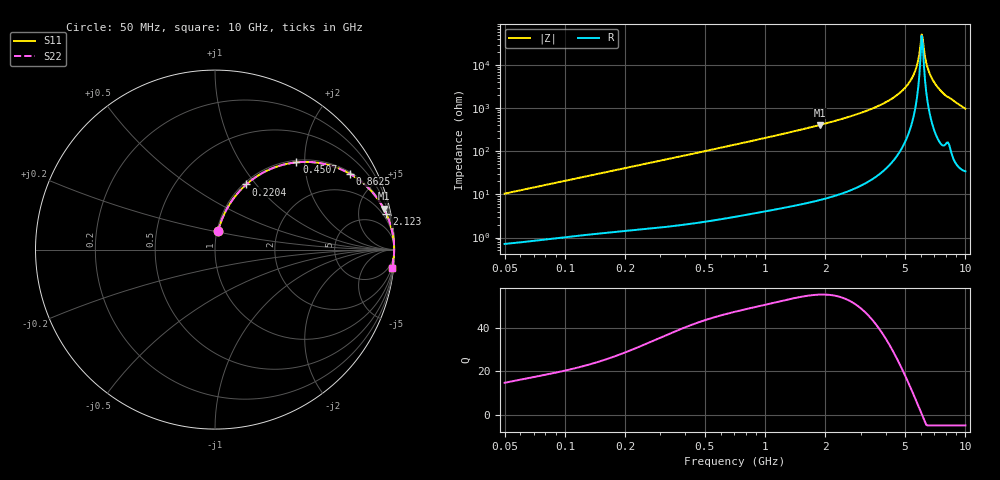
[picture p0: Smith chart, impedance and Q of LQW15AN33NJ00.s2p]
!Murata Part Number: LQW15AN33NJ00
!These Parameters are Measured in Series Mode Connection
!  o--[Z]--o
!Port1  Port2
!  o-------o
!Freq. Start=50[MHz] Stop=10[GHz], 401[Steps]
# Hz S RI R 50
!Freq.(Hz)	S 11(Real)	S 11(Imag)	S 21(Real)	S 21(Imag)	S 12(Real)	S 12(Imag)	S 22(Real)	S 22(Imag)
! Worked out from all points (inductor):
!   401 points, 50 MHz to 10 GHz, reference 50 ohm
!   read as one part in series: L = 33 nH near 51.34 MHz
!   highest Q = 55.3 at 1.884 GHz (marker M1), where L = 34.7 nH
!   self-resonance near 6.045 GHz
!   S11 on the Smith chart (normalised r, x): 50 MHz: 1.01, +0.21; 220.4 MHz: 1.03, +0.89; 450.7 MHz: 1.04, +1.82; 862.5 MHz: 1.07, +3.51; 2.123 GHz: 1.17, +9.53; 10 GHz: 2, -20
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5e7  0.0175 0.1015  0.9825 -0.1015  0.9825 -0.1015  0.0175 0.1015
1.214486e8  0.0673 0.2291  0.9327 -0.2291  0.9327 -0.2291  0.0673 0.2291
2.204238e8  0.1742 0.3631  0.8258 -0.3631  0.8258 -0.3631  0.1742 0.3631
2.949953e8  0.2678 0.4288  0.7322 -0.4288  0.7322 -0.4288  0.2678 0.4288
4.507103e8  0.4536 0.4861  0.5464 -0.4861  0.5464 -0.4861  0.4536 0.4861
7.071068e8  0.6686 0.4603  0.3314 -0.4603  0.3314 -0.4603  0.6686 0.4603
8.625288e8  0.7502 0.4229  0.2498 -0.4229  0.2498 -0.4229  0.7502 0.4229
1.717543e9  0.9276 0.2503  0.0724 -0.2503  0.0724 -0.2503  0.9276 0.2503
1.884411e9  0.9406 0.2276  0.0594 -0.2276  0.0594 -0.2276  0.9406 0.2276
2.122994e9  0.9545 0.1995  0.0455 -0.1995  0.0455 -0.1995  0.9545 0.1995
3.158828e9  0.9839 0.1157  0.0161 -0.1157  0.0161 -0.1157  0.9839 0.1157
4.171863e9  0.9938 0.0646  0.00621 -0.0646  0.00621 -0.0646  0.9938 0.0646
4.826234e9  0.9966 0.0393  0.00342 -0.0393  0.00342 -0.0393  0.9966 0.0393
5.365732e9  0.9977 0.0212  0.00226 -0.0212  0.00226 -0.0212  0.9977 0.0212
5.657692e9  0.9981 0.0121  0.00195 -0.0121  0.00195 -0.0121  0.9981 0.0121
5.965537e9  0.9982 0.003  0.00181 -0.003  0.00181 -0.003  0.9982 0.003
6.045081e9  0.9982 0.000712  0.0018 -0.000712  0.0018 -0.000712  0.9982 0.000712
6.207365e9  0.9982 -0.00388  0.00182 0.00388  0.00182 0.00388  0.9982 -0.00388
6.54512e9  0.998 -0.0132  0.00201 0.0132  0.00201 0.0132  0.998 -0.0132
7.086521e9  0.9973 -0.0275  0.00273 0.0275  0.00273 0.0275  0.9973 -0.0275
7.878683e9  0.9945 -0.0478  0.00554 0.0478  0.00554 0.0478  0.9945 -0.0478
1e10  0.9862 -0.1006  0.0138 0.1006  0.0138 0.1006  0.9862 -0.1006
